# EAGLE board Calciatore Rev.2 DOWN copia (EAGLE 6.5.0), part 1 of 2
Robot Calciatore SMD V2 Costruttori: Fabio Ricci Alessio Di Brigida
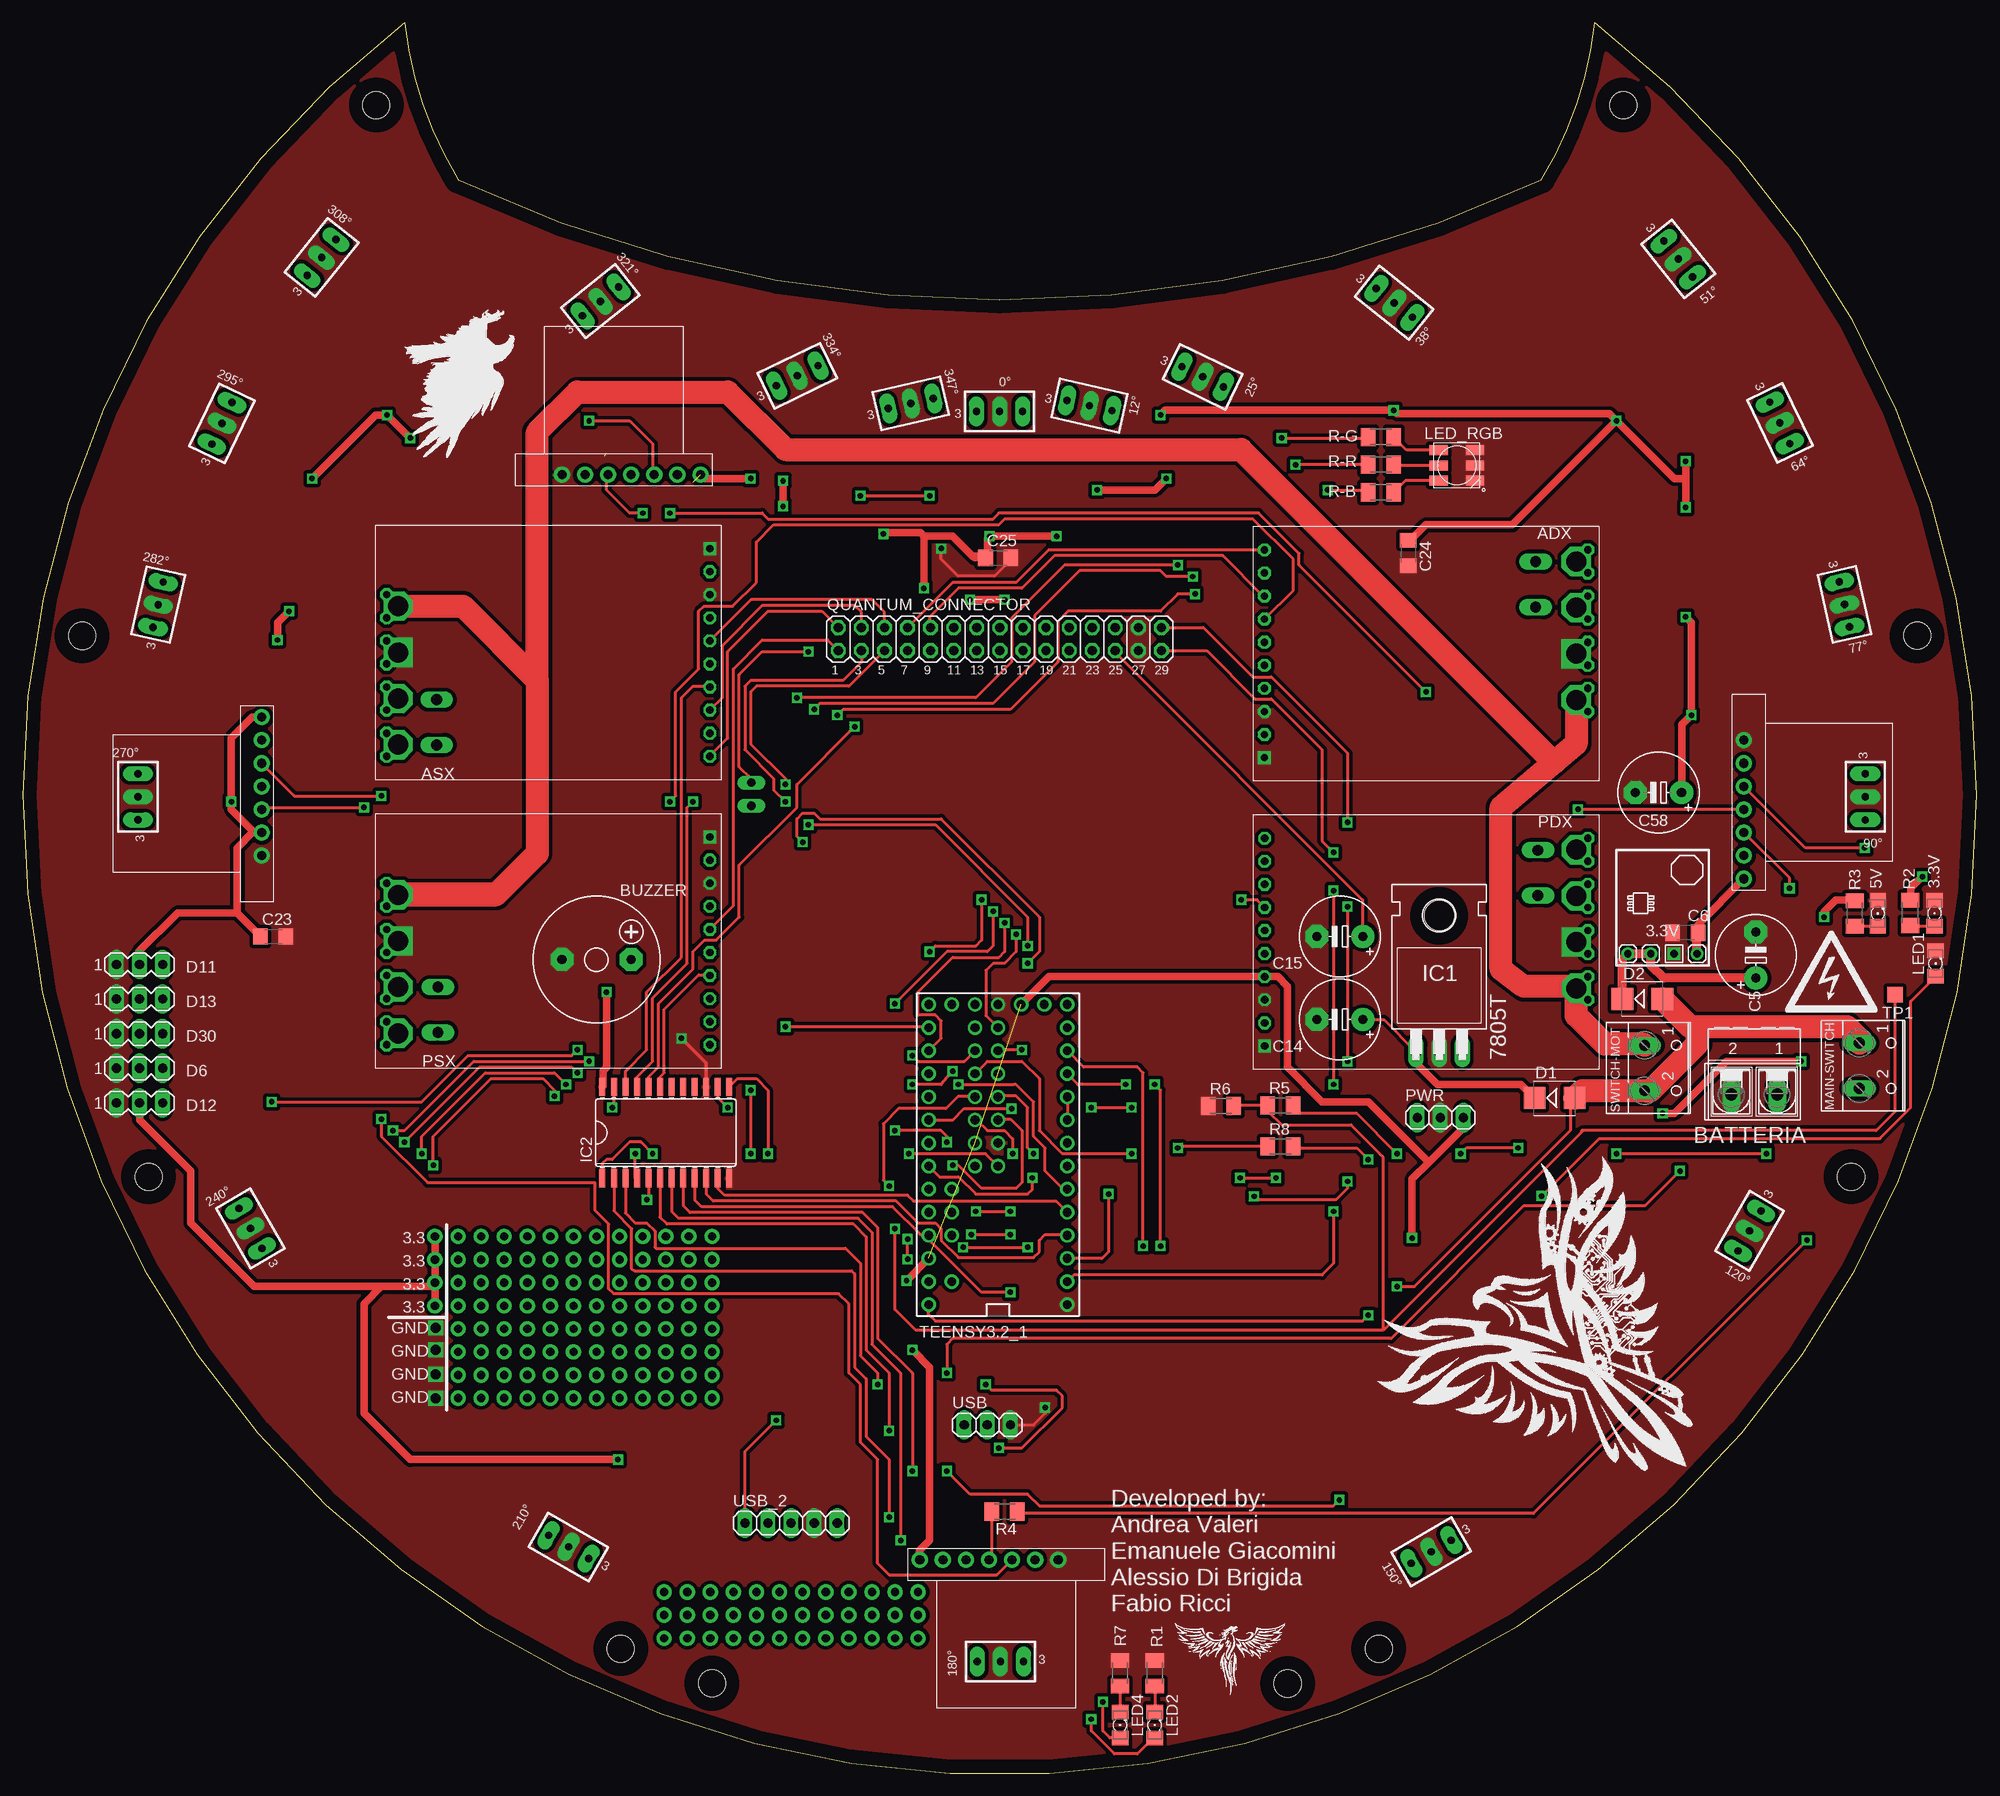
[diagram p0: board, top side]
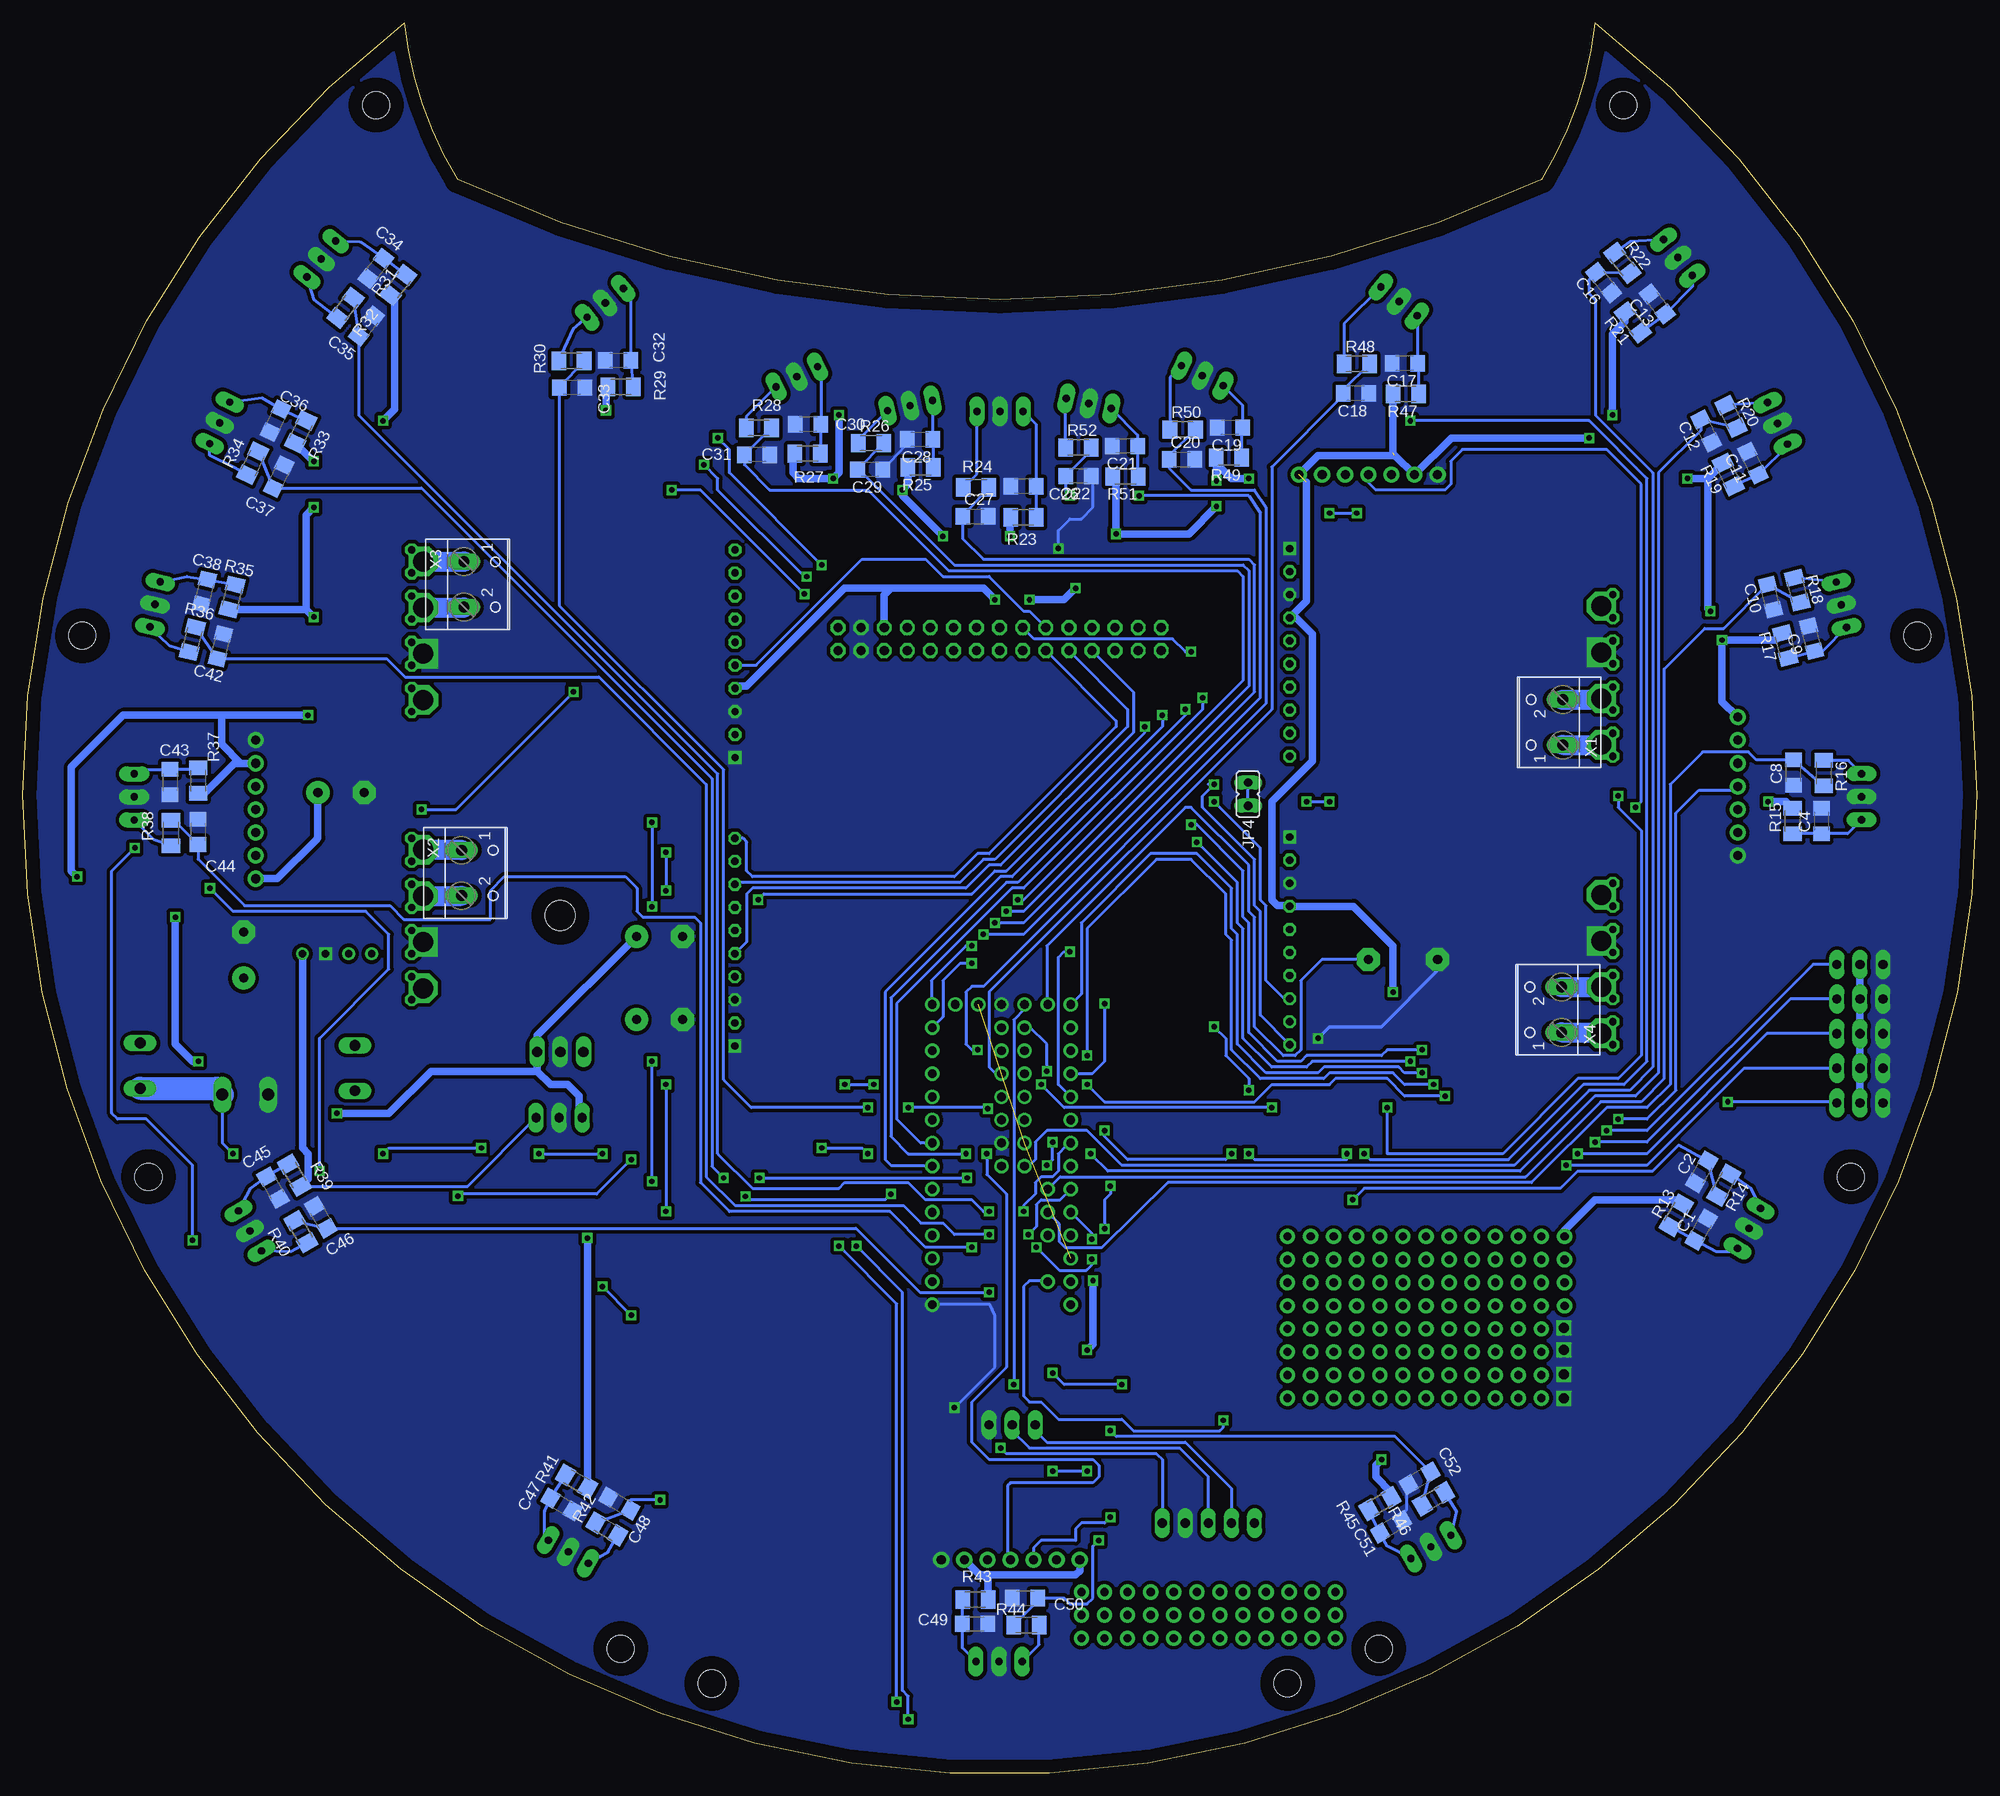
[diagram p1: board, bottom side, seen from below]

Size 214.99 x 192.6 mm. Coordinates in mm from the lower left corner, seen from the top.
Outline: 167.1,175.33 arc25 173,192.6 arc-25 167.1,175.33
Outline: 47.9,175.33 arc50 167.1,175.33
Outline: 47.9,175.33 arc-25 42,192.6 arc285 172.99,192.6
Copper layers (1*16): Top 0.035mm / dielectric 1.5mm / Bottom 0.035mm
Design rules "SparkFun *": minimum track width 8mil, minimum drill 20mil, track to track 8mil, track to pad 8mil, pad to pad 8mil, via to via 8mil, smd to smd 8mil, copper to edge 1.5mm, drill to drill 8mil, minimum pad ring 12mil, minimum via ring 10mil, stop-mask expansion 4mil, vias tented up to drill 25mil, thermal gap 0mil
Net classes: 0 default: width 0.254 mm, drill 0.254 mm, clearance 0.203 mm; 1 power: width 1.016 mm, drill 0.889 mm, clearance 0.508 mm; 2 gnd: width 0.864 mm, drill 0.406 mm, clearance 0.381 mm; 3 power usb: width 0.305 mm, drill 0.406 mm, clearance 0.203 mm
Holes 3 mm at 38.9,183.53 6.54,125.13 13.85,65.62 65.8,13.7 75.83,9.89 139.18,9.87 149.21,13.7 201.15,65.62 208.44,125.16 176.11,183.53

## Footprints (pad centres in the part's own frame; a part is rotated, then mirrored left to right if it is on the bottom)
TSOP4840 = drill 0.8 pad 1.676 long: GND 0,0; OUT -2.54,0; VCC 2.54,0
FKIT-LED-1206 = smd 1.6 x 1.803: A -1.422,0; C 1.422,0
MOTOR-SHIELD = drill 0.8 octagon: CS 29.21,-5.08; ENA/DIAGA 29.21,-10.16; ENB/DIAGB 29.21,-2.54; GND2 29.21,5.08; GNDMOT-2 -6.35,0; GNDMOT-3 -6.35,-2.54; INA 29.21,-12.7; INB 29.21,0; OUTA-2 -6.35,-10.16; OUTA-3 -6.35,-12.7; OUTB-2 -6.35,-5.08; OUTB-3 -6.35,-7.62; PWM 29.21,-7.62; VDD 29.21,2.54; VMOT-2 -6.35,5.08; VMOT-3 -6.35,2.54; VOUT 29.21,7.62 | drill 0.8 square: GND 29.21,10.16 | drill 2.2 square: GNDMOT-1 -5.08,-1.27 | drill 2.2 octagon: INMOT1 -5.08,-6.35; INMOT2 -5.08,-11.43; VMOT-1 -5.08,3.81
MB1010 = drill 1 pad 1.778: AN 2.54,-2.54; BW 7.62,-2.54; GND -7.62,-2.54; PW 5.08,-2.54; RX 0,-2.54; TX -2.54,-2.54; VCC -5.08,-2.54
AK500/2-H = drill 1.321 long: 1 -2.515,0; 2 2.515,0
F/CM12P = drill 1.016 pad 2.54 octagon: + 3.81,0; - -3.81,0
C1206 = smd 1.6 x 1.8: 1 -1.4,0; 2 1.4,0
E5-8,5 = drill 1.016 pad 2.54: + -2.54,0 | drill 1.016 pad 2.54 octagon: - 2.54,0
SMB = smd 2.4 x 2.4: A 2.2,0; C -2.2,0
MA03-1 = drill 1.016 long: 1 -2.54,0; 2 0,0; 3 2.54,0
TO220H = drill 1.118 long: 1 -2.54,-10.16; 2 0,-10.16; 3 2.54,-10.16 | hole 3.302: 0,4.826
SO24W = smd 0.66 x 2.032: 1 -6.985,-5.029; 2 -5.715,-5.029; 3 -4.445,-5.029; 4 -3.175,-5.029; 5 -1.905,-5.029; 6 -0.635,-5.029; 7 0.635,-5.029; 8 1.905,-5.029; 9 3.175,-5.029; 10 4.445,-5.029; 11 5.715,-5.029; 12 6.985,-5.029; 13 6.985,5.029; 14 5.715,5.029; 15 4.445,5.029; 16 3.175,5.029; 17 1.905,5.029; 18 0.635,5.029; 19 -0.635,5.029; 20 -1.905,5.029; 21 -3.175,5.029; 22 -4.445,5.029; 23 -5.715,5.029; 24 -6.985,5.029
JP1 = drill 0.914 long: 1 0,-1.27; 2 0,1.27
1206 = smd 1.6 x 1.803: A -1.422,0; C 1.422,0
RGBLED5050 = smd 2 x 1.1: 1 -2,1.7; 2 -2,0; 3 -2,-1.7; 4 2,-1.7; 5 2,0; 6 2,1.7
W237-102 = drill 1.194 long: 1 -2.5,-1.27; 2 2.5,-1.27
1X03 = drill 1.016 long: 1 -2.54,0; 2 0,0; 3 2.54,0
2X15 = drill 1.016 octagon: 1 -17.78,-1.27; 2 -17.78,1.27; 3 -15.24,-1.27; 4 -15.24,1.27; 5 -12.7,-1.27; 6 -12.7,1.27; 7 -10.16,-1.27; 8 -10.16,1.27; 9 -7.62,-1.27; 10 -7.62,1.27; 11 -5.08,-1.27; 12 -5.08,1.27; 13 -2.54,-1.27; 14 -2.54,1.27; 15 0,-1.27; 16 0,1.27; 17 2.54,-1.27; 18 2.54,1.27; 19 5.08,-1.27; 20 5.08,1.27; 21 7.62,-1.27; 22 7.62,1.27; 23 10.16,-1.27; 24 10.16,1.27; 25 12.7,-1.27; 26 12.7,1.27; 27 15.24,-1.27; 28 15.24,1.27; 29 17.78,-1.27; 30 17.78,1.27
M1206 = smd 1.6 x 2: 1 -1.4,0; 2 1.4,0
TEENSY3_ALL_PINS_&_PADS = drill 0.965: 0 -7.62,13.97; 1 -7.62,11.43; 2 -7.62,8.89; 3 -7.62,6.35; 3.3V 7.62,11.43; 3.3V1 -2.54,-16.51; 3.3V2 2.54,-1.27; 4 -7.62,3.81; 5 -7.62,1.27; 6 -7.62,-1.27; 7 -7.62,-3.81; 8 -7.62,-6.35; 9 -7.62,-8.89; 10 -7.62,-11.43; 11 -7.62,-13.97; 12 -7.62,-16.51; 13 7.62,-16.51; 14/A0 7.62,-13.97; 15/A1 7.62,-11.43; 16/A2 7.62,-8.89; 17/A3 7.62,-6.35; 18/A4 7.62,-3.81; 19/A5 7.62,-1.27; 20/A6 7.62,1.27; 21/A7 7.62,3.81; 22/A8 7.62,6.35; 23/A9 7.62,8.89; 24 0,-3.81; 25 0,-6.35; 26 0,-8.89; 27 0,-11.43; 28 0,-13.97; 29 2.54,-13.97; 30 2.54,-11.43; 31 2.54,-8.89; 32 2.54,-6.35; 33 2.54,-3.81; A10 5.08,6.35; A11 5.08,3.81; A12 0,1.27; A13 2.54,1.27; AGND 7.62,13.97; AREF 5.08,8.89; GND -7.62,16.51; GND1 0,-16.51; GND2 0,-1.27; PGM 2.54,-16.51; RESET/DAC 5.08,-16.51; VBAT -5.08,-16.51; VIN 7.62,16.51; VUSB 5.08,13.97
TP17SQ = smd 1.7 x 1.7: TP 0,0
ALIM_SWITCHING = drill 0.8 square: GND 1.27,-3.81 | drill 0.8: SHDN -3.81,-3.81; VIN -1.27,-3.81; VOUT 3.81,-3.81
1X05 = drill 1.016 long: 1 -5.08,0; 2 -2.54,0; 3 0,0; 4 2.54,0; 5 5.08,0

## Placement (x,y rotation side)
0°  effe  [TSOP4840]  107.47,149.84 180 top
3.3V  Power LED  [FKIT-LED-1206]  210.34,94.61 90 top
5V  Power LED  [FKIT-LED-1206]  204.11,94.61 90 top
12°  effe  [TSOP4840]  117.38,150.48 167.2 top
25°  effe  [TSOP4840]  129.82,153.65 154.2 top
38°  effe  [TSOP4840]  150.91,161.78 141.4 top
51°  effe  [TSOP4840]  182.15,166.6 128.6 top
64°  effe  [TSOP4840]  193.32,148.57 115.8 top
77°  effe  [TSOP4840]  200.44,128.6 102.8 top
90°  effe  [TSOP4840]  202.72,107.42 90 top
120°  effe  [TSOP4840]  190,59.67 60 top
150°  effe  [TSOP4840]  154.97,24.36 30 top
180°  effe  [TSOP4840]  107.57,12.27 0 top
210°  effe  [TSOP4840]  60.05,24.9 330 top
240°  effe  [TSOP4840]  25.06,59.94 300 top
270°  effe  [TSOP4840]  12.67,107.44 270 top
282°  effe  [TSOP4840]  14.9,128.57 257.2 top
295°  effe  [TSOP4840]  21.91,148.53 244.2 top
308°  effe  [TSOP4840]  32.88,166.77 231.4 top
321°  effe  [TSOP4840]  63.57,161.94 218.6 top
334°  effe  [TSOP4840]  85.21,153.76 205.8 top
347°  effe  [TSOP4840]  97.71,150.72 192.8 top
ADX  VHN5019  [MOTOR-SHIELD]  165.84,121.9 180 top
ASX  VHN5019  [MOTOR-SHIELD]  46.38,124.59 0 top
AX  MB1010  [MB1010]  66.95,145.41 0 top
BATTERIA  [AK500/2-H]  190.52,74.67 180 top
BUZZER  F/CM12P  [F/CM12P]  63.14,89.53 0 top
C1  [C1206]  30.32,59.81 60 bottom
C2  [C1206]  30.27,66.16 60 bottom
C4  [C1206]  17.06,104.77 90 bottom
C5  [E5-8,5]  190.69,90.02 90 top
C6  100n  [C1206]  182.94,92.46 180 top
C8  [C1206]  20.16,110.1 90 bottom
C9  [C1206]  18.18,124.83 104 bottom
C10  [C1206]  22.7,129.41 104 bottom
C11  [C1206]  24.63,144.14 116 bottom
C12  [C1206]  29.76,147.69 116 bottom
C13  [C1206]  35.15,161.66 128 bottom
C14  [E5-8,5]  144.92,82.92 180 top
C15  220uF  [E5-8,5]  144.92,92.07 180 top
C16  [C1206]  41.04,164 128 bottom
C17  [C1206]  62.93,155.11 180 bottom
C18  [C1206]  68.32,151.81 180 bottom
C19  470n  [C1206]  82.19,148.05 180 bottom
C20  470n  [C1206]  87.47,144.54 0 bottom
C21  [C1206]  93.72,146.02 180 bottom
C22  [C1206]  98.85,142.72 180 bottom
C23  100n  [C1206]  27.58,92.07 0 top
C24  100n  [C1206]  152.42,134.23 270 top
C25  100n  [C1206]  107.33,133.72 0 top
C26  470n  [C1206]  104.91,141.58 180 bottom
C27  470n  [C1206]  110.18,138.28 0 bottom
C28  [C1206]  116.28,146.74 180 bottom
C29  [C1206]  121.75,143.42 180 bottom
C30  [C1206]  128.57,148.42 180 bottom
C31  [C1206]  134.19,145.07 180 bottom
C32  [C1206]  149.48,155.43 180 bottom
C33  [C1206]  154.56,152.44 180 bottom
C34  [C1206]  176.13,165.58 232 bottom
C35  [C1206]  177.16,159.25 232 bottom
C36  [C1206]  187.16,148.82 244 bottom
C37  [C1206]  186.83,142.66 244 bottom
C38  [C1206]  195.02,129.99 256 bottom
C42  [C1206]  193.25,123.99 256 bottom
C43  [C1206]  198.8,109.04 270 bottom
C44  [C1206]  195.71,103.58 270 bottom
C45  [C1206]  187.46,64.43 300 bottom
C46  [C1206]  182.2,61.16 300 bottom
C47  [C1206]  155.71,29.57 330 bottom
C48  [C1206]  149.34,29.67 330 bottom
C49  [C1206]  110.22,16.43 0 bottom
C50  [C1206]  104.72,19.28 0 bottom
C51  [C1206]  64.44,27.12 30 bottom
C52  [C1206]  61.31,32.44 30 bottom
C58  220uF  [E5-8,5]  179.98,107.89 180 top
D1  M7  [SMB]  168.55,74.29 0 top
D2  M7  [SMB]  178.21,85.2 0 top
D6  [MA03-1]  12.86,77.56 0 top
D11  [MA03-1]  12.85,88.98 0 top
D12  [MA03-1]  12.86,73.75 0 top
D13  [MA03-1]  12.86,85.18 0 top
D30  [MA03-1]  12.86,81.37 0 top
DX  MB1010  [MB1010]  191.91,106.04 270 top
HIGHVOLTAGE  LOGO  [LOGOHV]  198.52,87.24 0 top
IC1  7805T  [TO220H]  155.85,89.53 0 top
IC2  4067D  [SO24W]  70.76,70.48 0 top
JP4  [JP1]  80.17,107.72 180 bottom
LED1  [1206]  210.47,89.09 90 top
LED2  [1206]  124.55,5.3 90 top
LED4  [1206]  120.74,5.3 90 top
LED_RGB  RGBLED5050  [RGBLED5050]  157.79,143.9 0 top
MAIN-SWITCH  [W237-102]  203.34,77.84 270 top
PDX  VHN5019  [MOTOR-SHIELD]  165.85,90.18 180 top
PSX  VHN5019  [MOTOR-SHIELD]  46.4,92.84 0 top
PWR  [1X03]  155.97,72.13 0 top
PX  MB1010  [MB1010]  106.32,20.95 180 top
QUANTUM_CONNECTOR  [2X15]  107.51,124.78 0 top
R1  330  [M1206]  124.55,11.01 270 top
R2  1K  [M1206]  207.66,94.67 90 top
R3  1K  [M1206]  201.57,94.61 90 top
R4  [M1206]  108.04,28.79 180 top
R5  10k  [M1206]  138.37,73.48 0 top
R6  3.3k  [M1206]  131.84,73.4 0 top
R7  330  [M1206]  120.74,11.01 270 top
R8  330  [M1206]  138.38,68.96 0 top
R13  [M1206]  33.06,61.39 60 bottom
R14  [M1206]  27.84,64.7 240 bottom
R15  [M1206]  20.26,104.77 90 bottom
R16  [M1206]  16.82,110.04 270 bottom
R17  [M1206]  21.07,124.07 104 bottom
R18  [M1206]  19.75,130.17 284 bottom
R19  [M1206]  27.32,142.87 116 bottom
R20  [M1206]  27.03,149.28 296 bottom
R21  [M1206]  37.84,159.63 128 bottom
R22  [M1206]  38.99,166.18 308 bottom
R23  1K  [M1206]  104.91,138.18 180 bottom
R24  33K  [M1206]  110.09,141.48 0 bottom
R25  [M1206]  116.22,143.67 180 bottom
R26  [M1206]  121.67,146.34 0 bottom
R27  [M1206]  128.63,145.2 180 bottom
R28  [M1206]  134,148.03 0 bottom
R29  [M1206]  149.19,152.54 180 bottom
R30  [M1206]  154.63,155.39 0 bottom
R31  [M1206]  173.68,163.74 232 bottom
R32  [M1206]  179.48,161.21 52 bottom
R33  [M1206]  184.4,147.59 244 bottom
R34  [M1206]  189.68,144.13 64 bottom
R35  [M1206]  191.96,129.41 256 bottom
R36  [M1206]  196.33,124.72 76 bottom
R37  [M1206]  195.67,109.2 270 bottom
R38  [M1206]  198.68,103.45 90 bottom
R39  [M1206]  185.09,65.8 300 bottom
R40  [M1206]  184.38,59.58 120 bottom
R41  [M1206]  154.06,32.11 330 bottom
R42  [M1206]  150.74,26.87 150 bottom
R43  [M1206]  110.18,19.11 0 bottom
R44  [M1206]  104.57,16.3 180 bottom
R45  [M1206]  65.66,29.66 30 bottom
R46  [M1206]  59.78,30.19 210 bottom
R47  [M1206]  62.83,151.76 180 bottom
R48  [M1206]  68.22,155.06 0 bottom
R49  1K  [M1206]  82.29,144.75 180 bottom
R50  33K  [M1206]  87.37,147.85 0 bottom
R51  [M1206]  93.67,142.67 180 bottom
R52  [M1206]  98.85,145.87 0 bottom
R-B  100  [M1206]  149.43,140.93 0 top
R-G  100  [M1206]  149.43,147.02 0 top
R-R  180  [M1206]  149.43,143.97 0 top
SWITCH-MOT  [W237-102]  179.72,77.59 270 top
SX  MB1010  [MB1010]  23.77,108.58 90 top
TEENSY3.2_1  TEENSY_3.1_ALL_PINS_AND_PADS  [TEENSY3_ALL_PINS_&_PADS]  107.31,68.07 180 top
TP1  PTR1TP17SQ  [TP17SQ]  205.99,85.65 90 top
U$5  [EAGLE-PLC-12MM]  54.05,161.02 180 top
U$8  PHOENIX_LOGHI  [PHOENIX_LOGHI]  126.48,8.4 0 top
U$10  ALIM  [ALIM_SWITCHING]  180.41,93.97 0 top
U$12  [PHOENIX]  168.93,48.38 45 top
USB  [1X03]  106.13,38.32 0 top
USB_2  [1X05]  84.54,27.52 0 top
X1  [W237-102]  46.82,115.63 90 bottom
X2  [W237-102]  165.45,99.06 270 bottom
X3  [W237-102]  165.18,130.8 270 bottom
X4  [W237-102]  46.96,84.01 90 bottom

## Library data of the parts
0° 12° 25° 38° 51° 64° 77° 90° 120° 150° 180° 210° 240° 270° 282° 295° 308° 321° 334° 347° = TSOP4840 IR
3.3V 5V = SparkFun-LED
ADX ASX PDX PSX = VHN5019; MOTOR: motor
AX DX PX SX = MaxSonar-mb1010
BATTERIA = con-ptr500; OC_FARNELL: unknown; OC_NEWARK: unknown
BUZZER = buzzer; OC_FARNELL: unknown; OC_NEWARK: unknown
C1 C2 C4 C8-C13 C16-C22 C26-C38 C42-C52 R4 R13-R52 = rcl
C5 C14 C15 C58 R1-R3 R5-R8 R-B R-G R-R = resistor
C6 C23-C25 = eagle-ltspice; SPICEMODEL: NONE; SPICEPREFIX: C
D1 D2 = diode
D6 D11-D13 D30 = con-lstb; OC_FARNELL: unknown; OC_NEWARK: unknown
HIGHVOLTAGE = Loghi
IC1 = linear
IC2 = 40xx
JP4 = jumper
LED1 LED2 LED4 LED_RGB = adafruit
MAIN-SWITCH SWITCH-MOT X1-X4 = con-wago-500; MPN: 237-102; OC_FARNELL: unknown; OC_NEWARK: 70K9898
PWR QUANTUM_CONNECTOR USB USB_2 = pinhead
TEENSY3.2_1 = Teensy_3_and_LC_Series_Boards_v1.1
TP1 = testpad
U$5 = logo
U$8 = loghi_phoenix
U$10 = Pololu switching alimentatore
U$12 = Phoenix

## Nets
3.3V [power usb]: ADX.VDD ASX.VDD AX.BW AX.VCC C6.1 C23.1 C24.1 C25.1 C58.+ D6.2 D11.2 D12.2 D13.2 D30.2 DX.BW DX.VCC IC2.24 PDX.VDD PSX.VDD PWR.3 PX.BW PX.VCC QUANTUM_CONNECTOR.26 R2.2 R13.2 R15.2 R17.2 R19.2 R21.2 R23.2 R25.2 R27.2 R29.2 R31.2 R33.2 R35.2 R37.2 R39.2 R41.2 R43.2 R45.2 R47.2 R49.2 R51.2 SX.BW SX.VCC TEENSY3.2_1.3.3V TEENSY3.2_1.3.3V1 TEENSY3.2_1.3.3V2 U$10.VOUT
5V: C15.+ IC1.3 PWR.1 QUANTUM_CONNECTOR.25 R3.2
AGND: TEENSY3.2_1.AGND
AREF: TEENSY3.2_1.AREF
BATLVL: R5.1 R6.2 TEENSY3.2_1.32 TP1.TP
BLUE(RGB): R-B.1 TEENSY3.2_1.5
BUZZER: BUZZER.+ TEENSY3.2_1.RESET/DAC
CS1: ASX.CS IC2.22
CS2: ADX.CS IC2.21
CS3: IC2.20 PDX.CS
CS4: IC2.19 PSX.CS
D+: USB.2 USB_2.3
D-: USB.1 USB_2.2
EXP-READ-1: IC2.1 TEENSY3.2_1.14/A0
EXPA: IC2.10 TEENSY3.2_1.2
EXPB: IC2.11 TEENSY3.2_1.3
EXPC: IC2.14 TEENSY3.2_1.4
EXPD: IC2.13 TEENSY3.2_1.24
GND [gnd]: 0°.GND 3.3V.C 5V.C 12°.GND 25°.GND 38°.GND 51°.GND 64°.GND 77°.GND 90°.GND 120°.GND 150°.GND 180°.GND 210°.GND 240°.GND 270°.GND 282°.GND 295°.GND 308°.GND 321°.GND 334°.GND 347°.GND ADX.GND ADX.GND2 ADX.GNDMOT-1 ASX.GND ASX.GND2 ASX.GNDMOT-1 AX.GND BATTERIA.2 BUZZER.- C1.2 C2.1 C4.2 C5.- C6.2 C8.1 C9.2 C10.1 C11.2 C12.1 C13.2 C14.- C15.- C16.1 C17.2 C18.1 C19.2 C20.2 C21.2 C22.1 C23.2 C24.2 C25.2 C26.2 C27.2 C28.2 C29.1 C30.2 C31.1 C32.2 C33.1 C34.2 C35.1 C36.2 C37.1 C38.2 C42.1 C43.2 C44.1 C45.2 C46.1 C47.2 C48.1 C49.2 C50.1 C51.2 C52.1 C58.- D6.1 D11.1 D12.1 D13.1 D30.1 DX.GND IC1.2 IC2.12 IC2.15 LED1.C LED_RGB.4 LED_RGB.5 LED_RGB.6 PDX.GND PDX.GND2 PDX.GNDMOT-1 PSX.GND PSX.GND2 PSX.GNDMOT-1 PWR.2 PX.GND QUANTUM_CONNECTOR.27 QUANTUM_CONNECTOR.28 R1.1 R6.1 R7.1 SX.GND TEENSY3.2_1.GND TEENSY3.2_1.GND1 TEENSY3.2_1.GND2 U$10.GND USB.3 USB_2.4
GREEN(RGB): R-G.1 TEENSY3.2_1.6
INA1-31-2: ASX.INA QUANTUM_CONNECTOR.2
INA2-32-2: ADX.INA QUANTUM_CONNECTOR.8
INA3-33-2: PDX.INA QUANTUM_CONNECTOR.11
INA4-34-2: PSX.INA QUANTUM_CONNECTOR.5
INB1-35-2: ASX.INB QUANTUM_CONNECTOR.6
INB2-36-2: ADX.INB QUANTUM_CONNECTOR.12
INB3-37-2: PDX.INB QUANTUM_CONNECTOR.7
INB4-38-2: PSX.INB QUANTUM_CONNECTOR.1
LED1: LED4.A TEENSY3.2_1.9
LED2: LED2.A TEENSY3.2_1.10
LED_ALIM: R8.1 TEENSY3.2_1.31
LINEA1: QUANTUM_CONNECTOR.15
LINEA2: QUANTUM_CONNECTOR.17
LINEA3: QUANTUM_CONNECTOR.19
LINEA4: QUANTUM_CONNECTOR.21
LINEA5: QUANTUM_CONNECTOR.23
LINEA6: QUANTUM_CONNECTOR.16
LINEA7: QUANTUM_CONNECTOR.18
LINEA8: QUANTUM_CONNECTOR.20
LINEA9: QUANTUM_CONNECTOR.22
LINEAANT: QUANTUM_CONNECTOR.24
MISO_12: D12.3 TEENSY3.2_1.12
MOSI_11: D11.3 TEENSY3.2_1.11
MOTORE1-1: ASX.INMOT2 X1.1
MOTORE1-2: ASX.INMOT1 X1.2
MOTORE2-1: PDX.INMOT2 X2.1
MOTORE2-2: PDX.INMOT1 X2.2
MOTORE3-1: ADX.INMOT2 X3.1
MOTORE3-2: ADX.INMOT1 X3.2
MOTORE4-1: PSX.INMOT2 X4.1
MOTORE4-2: PSX.INMOT1 X4.2
N$1: LED2.C R1.2
N$2: LED1.A R8.2
N$3: 0°.VCC C26.1 R23.1
N$4: 0°.OUT R24.1
N$6: 12°.VCC C28.1 R25.1
N$7: 12°.OUT R26.1
N$9: 240°.VCC C1.1 R13.1
N$12 [power usb]: PX.PW
N$13: 270°.VCC C4.1 R15.1
N$14: 282°.VCC C9.1 R17.1
N$15: 25°.OUT R28.1
N$16: 38°.OUT R30.1
N$17 [power]: C5.+ D2.C U$10.SHDN U$10.VIN
N$18: 51°.OUT R32.1
N$20: 25°.VCC C30.1 R27.1
N$24: 295°.VCC C11.1 R19.1
N$25: 308°.VCC C13.1 R21.1
N$26: 321°.VCC C17.1 R47.1
N$27: 64°.OUT R34.1
N$28: 38°.VCC C32.1 R29.1
N$34: 77°.OUT R36.1
N$35: 51°.VCC C34.1 R31.1
N$36: 120°.OUT R40.1
N$37: 64°.VCC C36.1 R33.1
N$38: 180°.OUT R44.1
N$39: 77°.VCC C38.1 R35.1
N$40: 90°.OUT R38.1
N$41: 90°.VCC C43.1 R37.1
N$42: 150°.OUT R42.1
N$43: 120°.VCC C45.1 R39.1
N$44: 210°.OUT R46.1
N$45: 150°.VCC C47.1 R41.1
N$51: 240°.OUT R14.1
N$52: 180°.VCC C49.1 R43.1
N$53: 270°.OUT R16.1
N$54: 210°.VCC C51.1 R45.1
N$56: 282°.OUT R18.1
N$57: 295°.OUT R20.1
N$60: 308°.OUT R22.1
N$64: 3.3V.A R2.1
N$65: 321°.OUT R48.1
N$67: LED_RGB.3 R-B.2
N$68: LED_RGB.1 R-G.2
N$69: LED4.C R7.2
N$81: LED_RGB.2 R-R.2
N$95: C14.+ D1.C IC1.1
N$97: 5V.A R3.1
N$190: 334°.VCC C19.1 R49.1
N$191: 347°.VCC C21.1 R51.1
N$200: AX.PW
N$201: 334°.OUT R50.1
N$202: 347°.OUT R52.1
N$215: DX.TX R4.1
N$233: DX.PW
N$366: SX.PW
NC: TEENSY3.2_1.7 TEENSY3.2_1.8
PALLA: QUANTUM_CONNECTOR.13
PROGRAM: TEENSY3.2_1.PGM USB_2.5
PWM1-2: ASX.PWM QUANTUM_CONNECTOR.4
PWM2-2: ADX.PWM QUANTUM_CONNECTOR.10
PWM3-2: PDX.PWM QUANTUM_CONNECTOR.9
PWM4-2: PSX.PWM QUANTUM_CONNECTOR.3
RED(RGB): R-R.1 TEENSY3.2_1.25
S1-A0: C27.1 R24.2 TEENSY3.2_1.15/A1
S2-A1: C29.2 R26.2 TEENSY3.2_1.16/A2
S3-A2: C31.2 R28.2 TEENSY3.2_1.17/A3
S4-A3: C33.2 R30.2 TEENSY3.2_1.18/A4
S5-A4: C35.2 R32.2 TEENSY3.2_1.19/A5
S6-A5: C37.2 R34.2 TEENSY3.2_1.20/A6
S7-A6: C42.2 R36.2 TEENSY3.2_1.21/A7
S8-A7: C44.2 R38.2 TEENSY3.2_1.22/A8
S9-A8: C46.2 IC2.9 R40.2 TEENSY3.2_1.23/A9
S10-A9: C48.2 IC2.8 R42.2
S11-A10: C50.2 IC2.7 R44.2
S12-A11: C52.2 IC2.6 R46.2
S13-A12: C2.2 IC2.5 R14.2
S14-A13: C8.2 R16.2 TEENSY3.2_1.A10
S15-A14: C10.2 R18.2 TEENSY3.2_1.A11
S16-A15: C12.2 R20.2 TEENSY3.2_1.A12
S17-A16: C16.2 R22.2 TEENSY3.2_1.A13
S18-A17: C18.2 R48.2 TEENSY3.2_1.26
S19-A18: C20.1 R50.2 TEENSY3.2_1.27
S20-A19: C22.2 R52.2 TEENSY3.2_1.28
SCK_13: D13.3 TEENSY3.2_1.13
SCL_29: D6.3 TEENSY3.2_1.29
SDA_30: D30.3 TEENSY3.2_1.30
SOLENOIDE: JP4.1 JP4.2 QUANTUM_CONNECTOR.14
TEENSY1-RX_TEENSY2-TX: QUANTUM_CONNECTOR.29 TEENSY3.2_1.0
TEENSY1-TX_TEENSY2-RX: QUANTUM_CONNECTOR.30 TEENSY3.2_1.1
TX1-RX2: PX.TX SX.RX
TX2-RX3: AX.RX SX.TX
TX3-RX4: AX.TX DX.RX
US-AX: AX.AN IC2.4
US-DX: DX.AN IC2.3
US-PX: IC2.2 PX.AN
US-SIGNAL: PX.RX R4.2 TEENSY3.2_1.33
US-SX: IC2.23 SX.AN
VBAT [power]: BATTERIA.1 MAIN-SWITCH.2 R5.2
VBATTEENSY: TEENSY3.2_1.VBAT
VIN [power]: D1.A D2.A MAIN-SWITCH.1 SWITCH-MOT.2 TEENSY3.2_1.VIN
VMOT [power]: ADX.VMOT-1 ASX.VMOT-1 PDX.VMOT-1 PSX.VMOT-1 SWITCH-MOT.1
VOUT: ASX.VOUT
VUSB: TEENSY3.2_1.VUSB USB_2.1

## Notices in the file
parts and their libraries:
SparkFun-LED: Licensing: Creative Commons ShareAlike 4.0 International - https://creativecommons.org/licenses/by-sa/4.0
